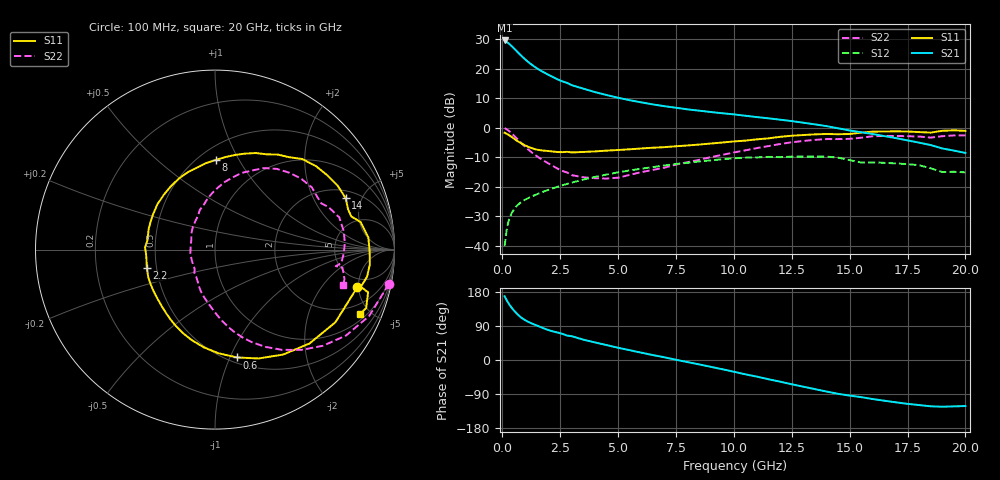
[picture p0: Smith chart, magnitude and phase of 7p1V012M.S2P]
! Infineon Technologies  Discrete & RF Semiconductors
! bfp620
! VCE =  1.0 V,  IC =  12 mA
! Common Emitter S-Parameters:  Sep 2002
# GHz  S  MA  R  50
!  f  S11  S21  S12  S22
! GHz  MAG  ANG  MAG  ANG  MAG  ANG  MAG  ANG
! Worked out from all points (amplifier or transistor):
!   59 points, 100 MHz to 20 GHz, reference 50 ohm
!   highest |S21| = 29.6 dB at 100 MHz (marker M1)
!   |S21| within 3 dB of that: start of sweep to 542.4 MHz
!   unconditionally stable (mu >= 1): 3.944 GHz to 10.36 GHz; 17.04 GHz to end of sweep
!   at 1 GHz: K = 0.55, MSG = 23.7 dB, |S12| = -24.4 dB
!   at 5.5 GHz: K = 1.04, MAG = 10.6 dB, |S12| = -14.5 dB
!   at 20 GHz: K = 1.43, MAG = -0.6 dB, |S12| = -15.1 dB
!   S11 on the Smith chart (normalised r, x): 100 MHz: 3.74, -4.81; 600 MHz: 0.55, -1.06; 2.2 GHz: 0.44, -0.11; 8 GHz: 0.60, +0.80; 14 GHz: 2.48, +3.67; 20 GHz: 1.33, -4.32
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0.1  0.8197 -14.9  30.12 168.2  0.0098 86.3  0.9873 -11.2
0.2  0.7836 -31.1  28.33 156.4  0.02 75.3  0.9351 -23.3
0.3  0.7423 -44.8  26.34 146.7  0.0284 68.9  0.8734 -33.2
0.4  0.6973 -57.0  24.25 138.2  0.0352 64.0  0.8056 -41.7
0.5  0.6533 -68.2  22.17 130.8  0.0411 60.0  0.7372 -49.3
0.6  0.6132 -78.5  20.23 124.1  0.046 56.7  0.6721 -56.2
0.8  0.5479 -96.6  16.88 112.9  0.054 52.1  0.5592 -67.9
0.9  0.5214 -104.2  15.49 108.5  0.0574 50.5  0.5121 -72.7
1.1  0.4777 -117.3  13.21 101.3  0.0634 48.2  0.4342 -80.6
1.3  0.4451 -128.2  11.47 95.8  0.0689 46.8  0.3739 -87.1
1.6  0.4172 -142.3  9.582 88.3  0.0773 45.2  0.3074 -96.1
2.2  0.3936 -164.8  7.165 75.2  0.0942 42.3  0.2226 -113.8
3  0.3804 172.7  5.252 62.8  0.1172 37.6  0.1566 -136.2
3.5  0.3879 161.7  4.59 53.7  0.1322 34.1  0.1444 -151.5
5  0.4182 132.9  3.22 32.3  0.1748 22.1  0.1419 158.5
7  0.4677 102.2  2.314 7.1  0.2287 4.3  0.2095 117.2
8  0.4993 89.6  2.044 -5.5  0.2538 -5.7  0.26 103.5
10.5  0.6044 61.4  1.593 -37.9  0.31 -33.6  0.4132 76.4
13.5  0.7707 27.5  1.139 -76.8  0.323 -67.9  0.6214 39.6
14  0.7822 21.5  1.063 -83.2  0.3232 -74.5  0.6414 32.7
17  0.8666 -5.5  0.666 -111.7  0.2478 -98.7  0.7242 2.9
20  0.8827 -24.0  0.373 -121.5  0.1748 -110.4  0.7419 -15.5
